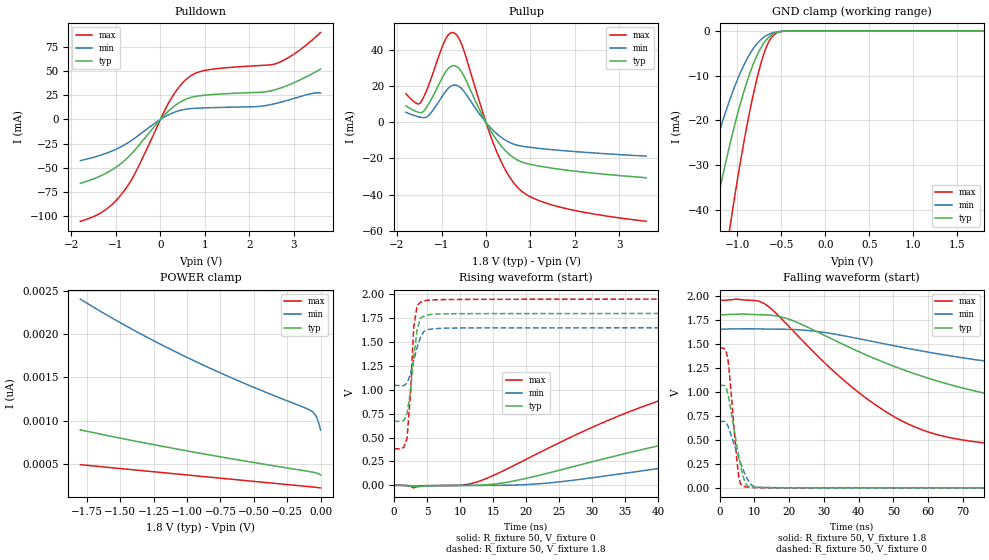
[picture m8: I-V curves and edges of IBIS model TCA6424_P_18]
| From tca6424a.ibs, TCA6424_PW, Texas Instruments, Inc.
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[Model]   TCA6424_P_18
Model_type  I/O
Vinl=0.495
Vinh=1.365
Enable   Active-Low
Vref =   0
Rref =   500
Cref =   50p
Vmeas =   0.9
| variable   typ   min   max
C_comp   3.65pF   2.87pF   4.06pF
| C_pullup   6.24pF   2.71pF   10.39pF
| C_pulldown   4.50pF   3.31pF   6.40pF
| C_tri-state   3.65pF   2.87pF   4.06pF
[Temperature Range]   40   100   -40
| Ambient temperature   25   85   -40
[Voltage range]   1.8   1.65   1.95
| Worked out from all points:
|   slope of the pulldown table from 0 to 0.27 V, typ, clamps not added: 22 ohm
|   slope of the pullup table from 0 to 0.27 V, typ, clamps not added: 25.1 ohm
|   GND clamp passes 1 mA (typ) near -0.61 V on its own axis
|   rising waveform, R_fixture 50, V_fixture 0: 20-80 % time 54.9ns typ, 67.1ns min, 34ns max; typ from 0 V to 1.06 V
|   falling waveform, R_fixture 50, V_fixture 1.8: 20-80 % time 57.7ns typ, 76.1ns min, 31.3ns max; typ from 1.8 V to 0.673 V
|   rising waveform, R_fixture 50, V_fixture 1.8: 20-80 % time 1.1ns typ, 1.41ns min, 773ps max; typ from 0.673 V to 1.8 V
|   falling waveform, R_fixture 50, V_fixture 0: 20-80 % time 3.14ns typ, 4.1ns min, 2.05ns max; typ from 1.06 V to 0 V
[GND Clamp]
| TCA6424_P_18
|   Voltage   I(typ)   I(min)   I(max)
-1.8V     -103.2mA   -70.78mA   -158.6mA
-1.495V   -66.41mA   -44.03mA   -105.9mA
-1.475V   -64.16mA   -42.41mA   -102.7mA
-1.275V   -42.97mA   -27.43mA   -71.16mA
-1.075V   -24.76mA   -14.94mA   -43.03mA
-965mV    -16.37mA   -9.431mA   -29.5mA
-860mV    -9.722mA   -5.298mA   -18.28mA
-760mV    -4.902mA   -2.55mA    -9.484mA
-675mV    -2.175mA   -1.137mA   -3.955mA
-585mV    -648.6uA   -385.3uA   -939.4uA
-455mV    -56.76uA   -45.75uA   -53.3uA
1.8V      377.4pA    1.171nA    151.4pA
[POWER Clamp]
| TCA6424_P_18
|   Voltage   I(typ)   I(min)   I(max)
-1.8V     896.4pA    2.402nA    495.2pA
-1.625V   839.9pA    2.24nA     469.1pA
-1.42V    776.4pA    2.062nA    438.7pA
-1.22V    716.9pA    1.899nA    409.1pA
-1.015V   658.2pA    1.742nA    378.8pA
-605mV    547.3pA    1.455nA    318.4pA
-80mV     415pA      1.124nA    241.3pA
-55mV     407.9pA    1.098nA    237.4pA
-35mV     400.6pA    1.058nA    234.2pA
-25mV     395.8pA    1.026nA    232.6pA
-15mV     389.6pA    982.1pA    230.9pA
-16.28fV  377.4pA    892.1pA    228.2pA
[Pulldown]
| TCA6424_P_18
|   Voltage   I(typ)   I(min)   I(max)
-1.8V     -65.79mA   -42.38mA   -105mA
-1.25V    -56.09mA   -35.39mA   -93.68mA
-815mV    -42.76mA   -26.44mA   -73.55mA
-545mV    -30.02mA   -18.21mA   -53.25mA
200mV     9.469mA    5.173mA    18.25mA
410mV     16.92mA    8.925mA    32.9mA
625mV     21.82mA    10.92mA    43.08mA
1.085V    25.45mA    12.08mA    51.29mA
2.18V     27.94mA    13.34mA    55.5mA
2.605V    31.03mA    16.64mA    57.72mA
3.06V     39.09mA    22.46mA    69.2mA
3.6V      51.88mA    27.15mA    89.64mA
[Pullup]
| TCA6424_P_18
|   Voltage   I(typ)   I(min)   I(max)
-1.8V     9.194mA    5.646mA    15.92mA
-1.475V   5.471mA    2.936mA    10.93mA
-1.295V   10.05mA    3.775mA    20.37mA
-920mV    27.6mA     16.84mA    45.72mA
-715mV    31.52mA    20.83mA    49.68mA
-520mV    26.88mA    18.01mA    41.62mA
-16.28fV  -48.38pA   -49.52pA   -51.71pA
230mV     -9.385mA   -5.982mA   -15.62mA
485mV     -16.82mA   -10.5mA    -28.47mA
740mV     -21.26mA   -12.85mA   -36.81mA
1.655V    -25.97mA   -15.47mA   -46.96mA
3.6V      -30.68mA   -18.69mA   -54.88mA
[Ramp]
| TCA6424_P_18
| variable   typ   min   max
dV/dt_r   0.65/5.51E-08   0.42/6.72E-08   0.89/3.42E-08
dV/dt_f   0.68/5.78E-08   0.36/7.62E-08   0.95/3.15E-08
R_load = 50
[Rising Waveform]
| TCA6424_P_18
R_fixture =   50
C_fixture =   0
L_fixture =   0
V_fixture =   0
V_fixture_min = 0
V_fixture_max = 0
|   Time   V(typ)   V(min)   V(max)
0s        1.475nV    11.41nV    451.1pV
12.5ns    697.6uV    -973.9uV   34.1mV
19ns      57.45mV    4.9mV      236.7mV
35ns      332.6mV    127.2mV    753.4mV
52ns      579.1mV    281.4mV    1.123V
66.5ns    730.3mV    385.9mV    1.296V
85.5ns    863.8mV    485.6mV    1.387V
121ns     989.2mV    593.1mV    1.436V
174ns     1.045V     656.7mV    1.449V
520ns     1.062V     686mV      1.451V
[Falling Waveform]
| TCA6424_P_18
R_fixture =   50
C_fixture =   0
L_fixture =   0
V_fixture =   1.8
V_fixture_min = 1.65
V_fixture_max = 1.95
|   Time   V(typ)   V(min)   V(max)
0s        1.8V       1.65V      1.95V
13.5ns    1.799V     1.652V     1.901V
21ns      1.74V      1.647V     1.64V
36ns      1.485V     1.58V      1.111V
52.5ns    1.233V     1.462V     695.4mV
64.5ns    1.092V     1.384V     536.5mV
81ns      948.1mV    1.297V     450.8mV
118ns     775.5mV    1.172V     398.5mV
172.5ns   697.9mV    1.092V     385.7mV
520ns     673.2mV    1.049V     383.8mV
[Rising Waveform]
| TCA6424_P_18
R_fixture =   50
C_fixture =   0
L_fixture =   0
V_fixture =   1.8
V_fixture_min = 1.65
V_fixture_max = 1.95
|   Time   V(typ)   V(min)   V(max)
0s        673.1mV    1.049V     383.8mV
1.5ns     677.8mV    1.044V     398.5mV
2ns       754.5mV    1.072V     498.9mV
2.5ns     988.4mV    1.166V     965.7mV
3ns       1.337V     1.31V      1.657V
3.5ns     1.625V     1.443V     1.88V
4ns       1.749V     1.547V     1.918V
4.5ns     1.771V     1.609V     1.931V
6ns       1.792V     1.639V     1.942V
520ns     1.8V       1.65V      1.95V
[Falling Waveform]
| TCA6424_P_18
R_fixture =   50
C_fixture =   0
L_fixture =   0
V_fixture =   0
V_fixture_min = 0
V_fixture_max = 0
|   Time   V(typ)   V(min)   V(max)
0s        1.062V     686.1mV    1.451V
1.5ns     1.061V     690.6mV    1.444V
2.5ns     962.4mV    636.2mV    1.314V
4.5ns     538mV      418mV      477.3mV
5.5ns     334.7mV    313mV      126.6mV
6ns       242.8mV    263mV      43.51mV
7ns       92.71mV    170.3mV    14.96mV
8.5ns     13.02mV    59.93mV    6.022mV
19.5ns    958.6uV    969.2uV    873.9uV
520ns     97.42nV    333.5nV    51.84nV
